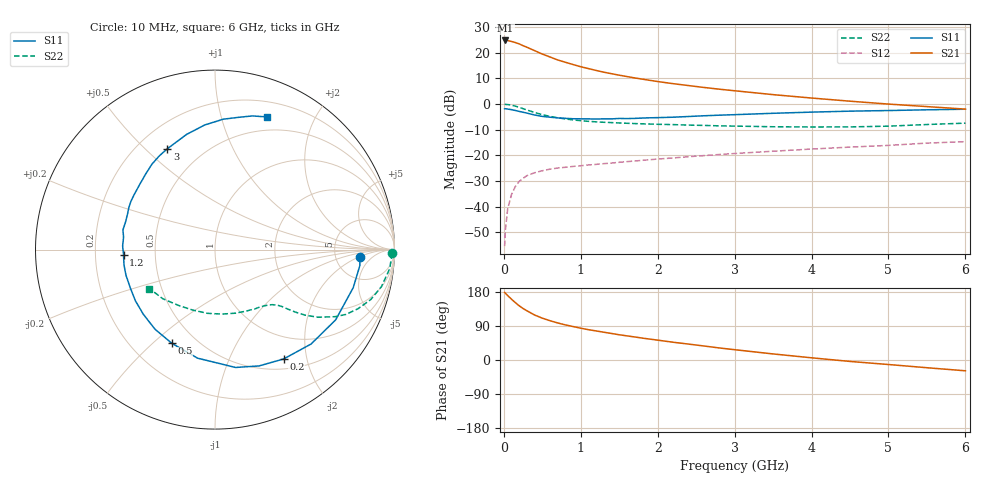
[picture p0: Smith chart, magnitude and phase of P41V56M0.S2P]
! SIEMENS Small Signal Semiconductors
! BFP182
! Si NPN RF Bipolar Junction Transistor in SOT143
! VCE = 1.5 V  IC = 6 mA
! Common Emitter S-Parameters:  March  1996
# GHz  S  MA  R  50
!  f  S11  S21  S12  S22
! GHz  MAG  ANG  MAG  ANG  MAG  ANG  MAG  ANG
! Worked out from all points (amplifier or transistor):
!   36 points, 10 MHz to 6 GHz, reference 50 ohm
!   highest |S21| = 24.8 dB at 20 MHz (marker M1)
!   |S21| within 3 dB of that: start of sweep to 326.8 MHz
!   unconditionally stable (mu >= 1): 1.384 GHz to 5.621 GHz
!   at 250 MHz: K = 0.24, MSG = 25.9 dB, |S12| = -28.9 dB
!   at 1.4 GHz: K = 1.01, MAG = 16.9 dB, |S12| = -23.0 dB
!   at 6 GHz: K = 0.96, MSG = 6.3 dB, |S12| = -14.6 dB
!   S11 on the Smith chart (normalised r, x): 10 MHz: 8.87, -2.24; 200 MHz: 0.64, -1.62; 500 MHz: 0.37, -0.58; 1.2 GHz: 0.32, -0.03; 3 GHz: 0.32, +0.59; 6 GHz: 0.35, +1.41
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0.01  0.8085 -3.1  17.29 178.1  0.0017 82.0  0.9875 -1.2
0.02  0.8119 -6.3  17.37 176.5  0.0035 88.7  0.9845 -2.5
0.05  0.7988 -15.4  17.32 169.9  0.0091 84.2  0.9787 -6.3
0.1  0.7779 -30.2  16.6 160.4  0.0173 74.1  0.9505 -12.5
0.15  0.7505 -44.5  15.8 151.3  0.0248 67.3  0.9112 -17.8
0.2  0.7193 -57.9  14.89 143.0  0.0311 61.8  0.8628 -22.4
0.25  0.6932 -69.2  13.73 135.9  0.0357 57.1  0.8145 -26.3
0.3  0.6666 -80.1  12.82 129.9  0.0403 53.0  0.7682 -29.1
0.4  0.6127 -99.1  10.99 118.7  0.0459 46.9  0.6865 -33.3
0.5  0.5748 -114.8  9.431 110.4  0.0502 42.4  0.6219 -36.0
0.6  0.5552 -127.1  8.274 103.7  0.0539 39.8  0.575 -37.6
0.7  0.5378 -138.0  7.248 97.8  0.0567 38.2  0.5409 -38.7
0.9  0.5176 -156.1  5.896 88.3  0.0609 36.3  0.4914 -40.3
1.1  0.5141 -170.5  4.915 80.0  0.065 35.5  0.4611 -42.1
1.2  0.5105 -176.7  4.522 76.7  0.0668 35.2  0.4501 -43.1
1.7  0.526 157.9  3.234 60.8  0.0776 35.4  0.4168 -48.6
2.2  0.5547 139.2  2.5 46.9  0.0892 35.0  0.3981 -56.3
3  0.6215 115.3  1.818 27.2  0.1087 32.2  0.3722 -72.1
3.5  0.6612 103.8  1.527 16.0  0.1205 29.7  0.3614 -83.8
4.5  0.7279 86.4  1.138 -3.8  0.1449 24.1  0.359 -110.2
5.5  0.7733 74.4  0.893 -20.4  0.1735 17.9  0.3995 -136.8
6  0.7939 68.6  0.797 -28.5  0.1853 13.3  0.4249 -149.3
